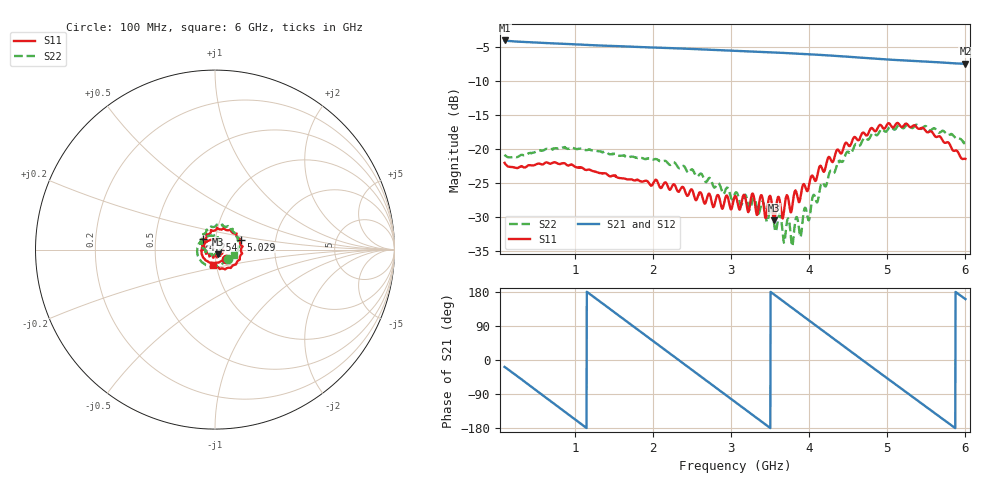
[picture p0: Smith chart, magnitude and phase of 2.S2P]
!Agilent Technologies,E5071C,MY46316741,A.11.02
!Date: Thu Dec 16 09:43:26 2021
!Data & Calibration Information:
!Freq	S11:SOLT4(ON)	S21:SOLT4(ON)	S12:SOLT4(ON)	S22:SOLT4(ON)
!PortZ  Port1:50+j0  Port2:50+j0
!Above PortZ is port z conversion or system Z0 setting when saving the data.
!When reading, reference impedance value at option line is always used.
# Hz S dB R 50
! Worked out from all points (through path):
!   1593 points, 100 MHz to 6 GHz, reference 50 ohm
!   highest |S21| = -4.10 dB at 100 MHz (marker M1); lowest = -7.5 dB at 6 GHz (marker M2)
!   group delay of S21, straight-line fit = 425 ps
!   lowest |S11| = -30.4 dB at 3.55 GHz (marker M3), VSWR 1.06, Z = 51.4 - j2.69 ohm
!   |S11| at or under -10 dB: start of sweep to end of sweep
!   |S22| runs from -34.2 to -16.4 dB; largest |S21 - S12| = 0.0034
!   S11 on the Smith chart (normalised r, x): 100 MHz: 1.12, -0.11; 4.254 GHz: 0.87, +0.10; 5.029 GHz: 1.32, +0.15; 6 GHz: 0.96, -0.16
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1e8  -22.03 -39.4  -4.10 -18.2  -4.11 -18.2  -20.83 -34.8
3.668342e8  -22.69 -84.5  -4.33 -58.8  -4.34 -58.8  -20.91 -78.3
5.817839e8  -22.28 -121.3  -4.45 -92.1  -4.46 -92.1  -20.25 -112.8
1.085804e9  -22.70 170.0  -4.72 -169.8  -4.72 -169.7  -19.93 -175.3
1.334108e9  -23.53 145.1  -4.85 152.2  -4.86 152.3  -20.39 162.4
1.615766e9  -24.31 123.8  -4.96 109.1  -4.97 109.1  -20.95 142.2
2.067902e9  -25.05 95.3  -5.16 39.9  -5.17 40.0  -21.62 110.7
2.482977e9  -25.98 57.5  -5.34 -23.7  -5.35 -23.7  -23.10 76.7
2.77946e9  -28.46 37.2  -5.48 -69.1  -5.49 -69.0  -25.60 60.4
3.05e9  -26.91 15.4  -5.62 -110.5  -5.63 -110.4  -26.55 41.1
3.442839e9  -30.12 -39.2  -5.80 -170.6  -5.81 -170.4  -29.87 13.6
3.49843e9  -26.87 -49.0  -5.83 -179.1  -5.84 -178.9  -28.86 -9.2
3.550314e9  -30.43 -60.2  -5.85 172.9  -5.86 173.1  -30.94 -2.0
3.783794e9  -28.38 -129.0  -6.00 137.1  -6.00 137.3  -34.23 -70.9
4.035804e9  -23.88 -179.0  -6.15 98.5  -6.15 98.7  -27.48 -147.5
4.25446e9  -21.16 139.8  -6.30 65.0  -6.31 65.2  -23.64 173.2
4.636181e9  -18.67 74.1  -6.61 6.8  -6.61 7.0  -19.54 123.6
5.017902e9  -16.22 21.5  -6.90 -51.1  -6.90 -50.9  -16.95 74.1
5.02902e9  -16.28 21.2  -6.91 -52.8  -6.91 -52.6  -16.80 73.7
5.432977e9  -16.97 -34.5  -7.18 -113.8  -7.17 -113.5  -17.06 32.1
5.722048e9  -18.98 -68.8  -7.36 -157.5  -7.34 -157.1  -17.38 6.2
6e9  -21.45 -98.0  -7.50 160.7  -7.50 161.0  -19.11 -15.8
